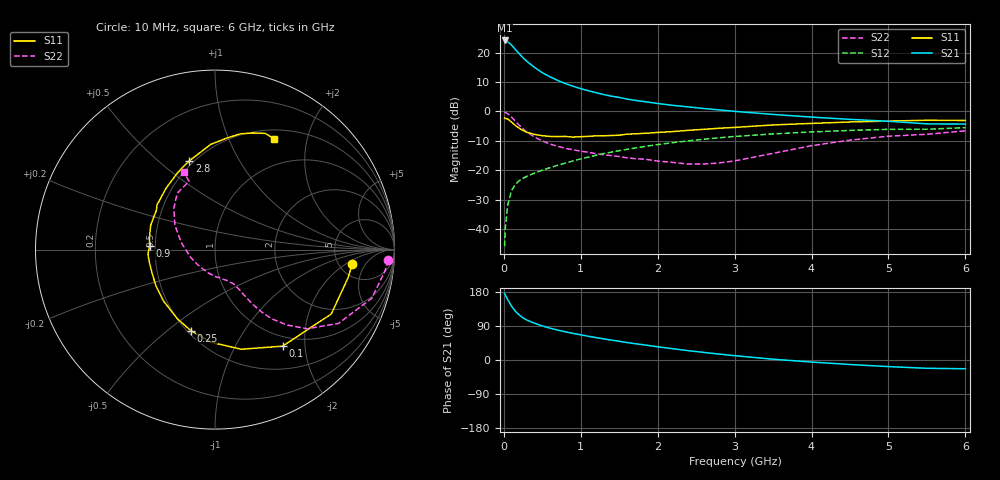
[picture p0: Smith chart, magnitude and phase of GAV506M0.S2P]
! Infineon Technologies  Discrete & RF Semiconductors
! BF775
! Si NPN RF Bipolar Junction Transistor in SOT23
! VCE = 0.5 V  IC = 6 mA
! Common Emitter S-Parameters:  May  1996
# GHz  S  MA  R  50
!  f  S11  S21  S12  S22
! GHz  MAG  ANG  MAG  ANG  MAG  ANG  MAG  ANG
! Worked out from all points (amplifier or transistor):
!   36 points, 10 MHz to 6 GHz, reference 50 ohm
!   highest |S21| = 24.1 dB at 10 MHz (marker M1)
!   |S21| within 3 dB of that: start of sweep to 147.1 MHz
!   unconditionally stable (mu >= 1): 550.7 MHz to end of sweep
!   at 250 MHz: K = 0.61, MSG = 20.5 dB, |S12| = -22.7 dB
!   at 1.4 GHz: K = 1.24, MAG = 6.5 dB, |S12| = -13.9 dB
!   at 6 GHz: K = 1.08, MAG = -1.2 dB, |S12| = -5.5 dB
!   S11 on the Smith chart (normalised r, x): 10 MHz: 6.57, -2.62; 100 MHz: 0.84, -1.59; 250 MHz: 0.52, -0.60; 900 MHz: 0.47, +0.02; 2.8 GHz: 0.47, +0.64; 6 GHz: 0.61, +1.48
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0.01  0.7685 -6.1  16.04 175.9  0.0051 87.1  0.9662 -3.5
0.02  0.7578 -12.0  15.93 171.3  0.0105 80.4  0.9544 -7.2
0.05  0.7405 -29.0  15.23 159.4  0.0254 75.3  0.9142 -17.3
0.1  0.6567 -55.0  13.39 142.1  0.0449 63.9  0.8008 -30.9
0.15  0.574 -75.3  11.24 128.5  0.0571 56.4  0.6774 -40.6
0.2  0.5168 -92.3  9.558 118.9  0.0662 52.3  0.5831 -46.2
0.25  0.4709 -106.7  8.141 111.1  0.073 50.2  0.5031 -50.4
0.3  0.4393 -118.3  7.066 105.4  0.0786 49.1  0.4437 -52.9
0.4  0.4053 -135.3  5.57 97.0  0.0893 49.1  0.3665 -55.6
0.5  0.3855 -148.9  4.542 89.9  0.0999 49.6  0.3143 -56.9
0.6  0.374 -160.0  3.861 84.0  0.1102 50.6  0.278 -58.2
0.7  0.3725 -169.2  3.359 78.9  0.121 51.2  0.2537 -59.0
0.9  0.3649 177.0  2.667 70.3  0.144 51.5  0.2219 -61.1
1.1  0.3757 164.5  2.239 62.6  0.167 51.4  0.201 -65.0
1.3  0.3842 154.7  1.928 55.7  0.1913 50.4  0.1825 -69.5
1.6  0.4094 142.1  1.618 46.1  0.2256 48.2  0.1625 -78.8
2.2  0.4531 122.3  1.262 29.7  0.2937 41.7  0.1353 -106.7
2.8  0.5157 106.0  1.058 15.6  0.3555 33.9  0.1325 -149.8
3.5  0.5869 92.3  0.886 2.1  0.4134 24.0  0.1929 167.9
4.5  0.6595 77.8  0.73 -11.9  0.4741 10.6  0.3239 135.1
5.5  0.7054 66.6  0.612 -21.9  0.4963 -2.2  0.4072 110.8
6  0.6996 62.0  0.607 -23.1  0.5282 -5.8  0.4662 111.9
